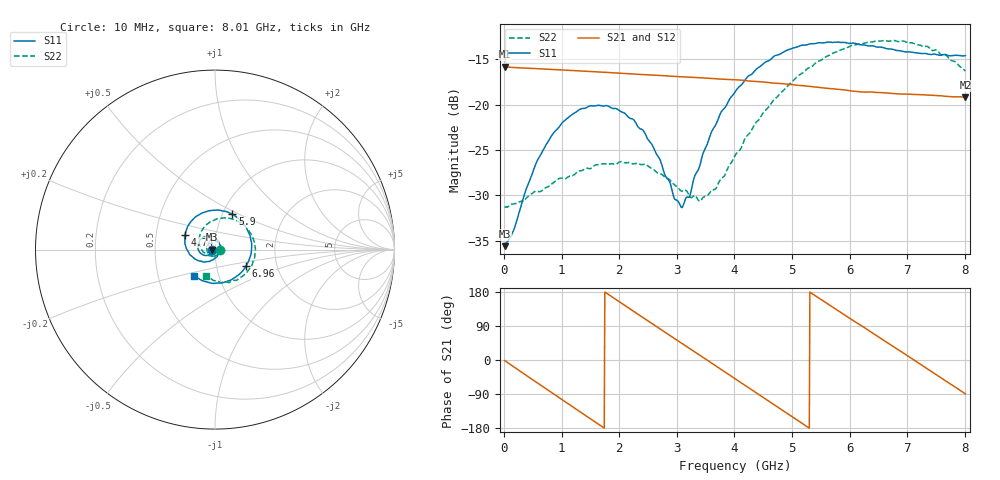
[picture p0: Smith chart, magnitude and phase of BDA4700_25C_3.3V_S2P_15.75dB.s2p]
!Agilent Technologies,E5071B,MY42404982,A.09.10
!Date: Mon Oct 20 18:09:39 2025
!Data & Calibration Information:
!Freq	S11:SOLT2(ON)	S21:SOLT2(ON)	S12:SOLT2(ON)	S22:SOLT2(ON)
# Hz S RI R 50
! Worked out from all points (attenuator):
!   801 points, 10 MHz to 8.01 GHz, reference 50 ohm
!   highest |S21| = -15.84 dB at 10 MHz (marker M1); lowest = -19.2 dB at 8.01 GHz (marker M2)
!   lowest |S11| = -35.6 dB at 10 MHz (marker M3), VSWR 1.03, Z = 48.4 - j0.109 ohm
!   |S11| at or under -10 dB: start of sweep to end of sweep
!   |S22| runs from -31.3 to -12.9 dB; largest |S21 - S12| = 0.0019
!   S11 on the Smith chart (normalised r, x): 10 MHz: 0.97, -0.00; 4.74 GHz: 0.70, +0.12; 5.9 GHz: 1.11, +0.46; 6.96 GHz: 1.39, -0.26; 8.01 GHz: 0.76, -0.23
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1e7  -0.0165 -0.00112  0.1613 -0.00351  0.1613 -0.00368  0.0274 -0.000994
1.6e8  -0.0175 -0.00987  0.1529 -0.0469  0.1529 -0.0469  0.0272 -0.00802
5.3e8  -0.0345 -0.0293  0.0895 -0.13  0.0894 -0.1301  0.0161 -0.029
7.3e8  -0.0503 -0.0329  0.0375 -0.1521  0.0376 -0.1521  0.00257 -0.0348
1.03e9  -0.077 -0.0234  -0.0452 -0.1482  -0.0452 -0.1482  -0.0196 -0.0338
1.35e9  -0.0949 0.00485  -0.1169 -0.0988  -0.1169 -0.0988  -0.0404 -0.0154
2.08e9  -0.0519 0.0737  -0.1226 0.0836  -0.1226 0.0836  -0.0253 0.0405
2.42e9  -0.00863 0.0713  -0.053 0.1362  -0.0529 0.1362  0.00414 0.0465
2.68e9  0.0178 0.0482  0.0128 0.1442  0.0125 0.1441  0.0227 0.0351
2.96e9  0.0282 0.0108  0.0783 0.1195  0.0782 0.1193  0.033 0.0148
3.1e9  0.0256 -0.00933  0.105 0.0959  0.1042 0.0965  0.0333 0.00169
3.23e9  0.0181 -0.026  0.123 0.0698  0.1231 0.0696  0.0299 -0.00823
3.42e9  -0.00167 -0.049  0.138 0.0253  0.1381 0.0253  0.0185 -0.0232
3.75e9  -0.0552 -0.0689  0.1273 -0.0537  0.1274 -0.0537  -0.0124 -0.0362
4.01e9  -0.1023 -0.0571  0.0893 -0.1038  0.0894 -0.1035  -0.0426 -0.0301
4.74e9  -0.1675 0.0838  -0.072 -0.1094  -0.0715 -0.1098  -0.0871 0.0668
5.35e9  -0.0642 0.2066  -0.125 0.0108  -0.125 0.01  -0.00864 0.162
5.9e9  0.0964 0.1975  -0.0602 0.1042  -0.0605 0.1039  0.1265 0.1583
6.68e9  0.2024 -0.00868  0.0842 0.079  0.0845 0.0789  0.2229 -0.0211
6.96e9  0.1725 -0.0917  0.1099 0.0309  0.1099 0.0302  0.2006 -0.0961
7.48e9  0.0404 -0.1852  0.0903 -0.0665  0.0905 -0.0667  0.0823 -0.1818
8.01e9  -0.1151 -0.1462  0.000852 -0.1099  0.00122 -0.1099  -0.0474 -0.1455
